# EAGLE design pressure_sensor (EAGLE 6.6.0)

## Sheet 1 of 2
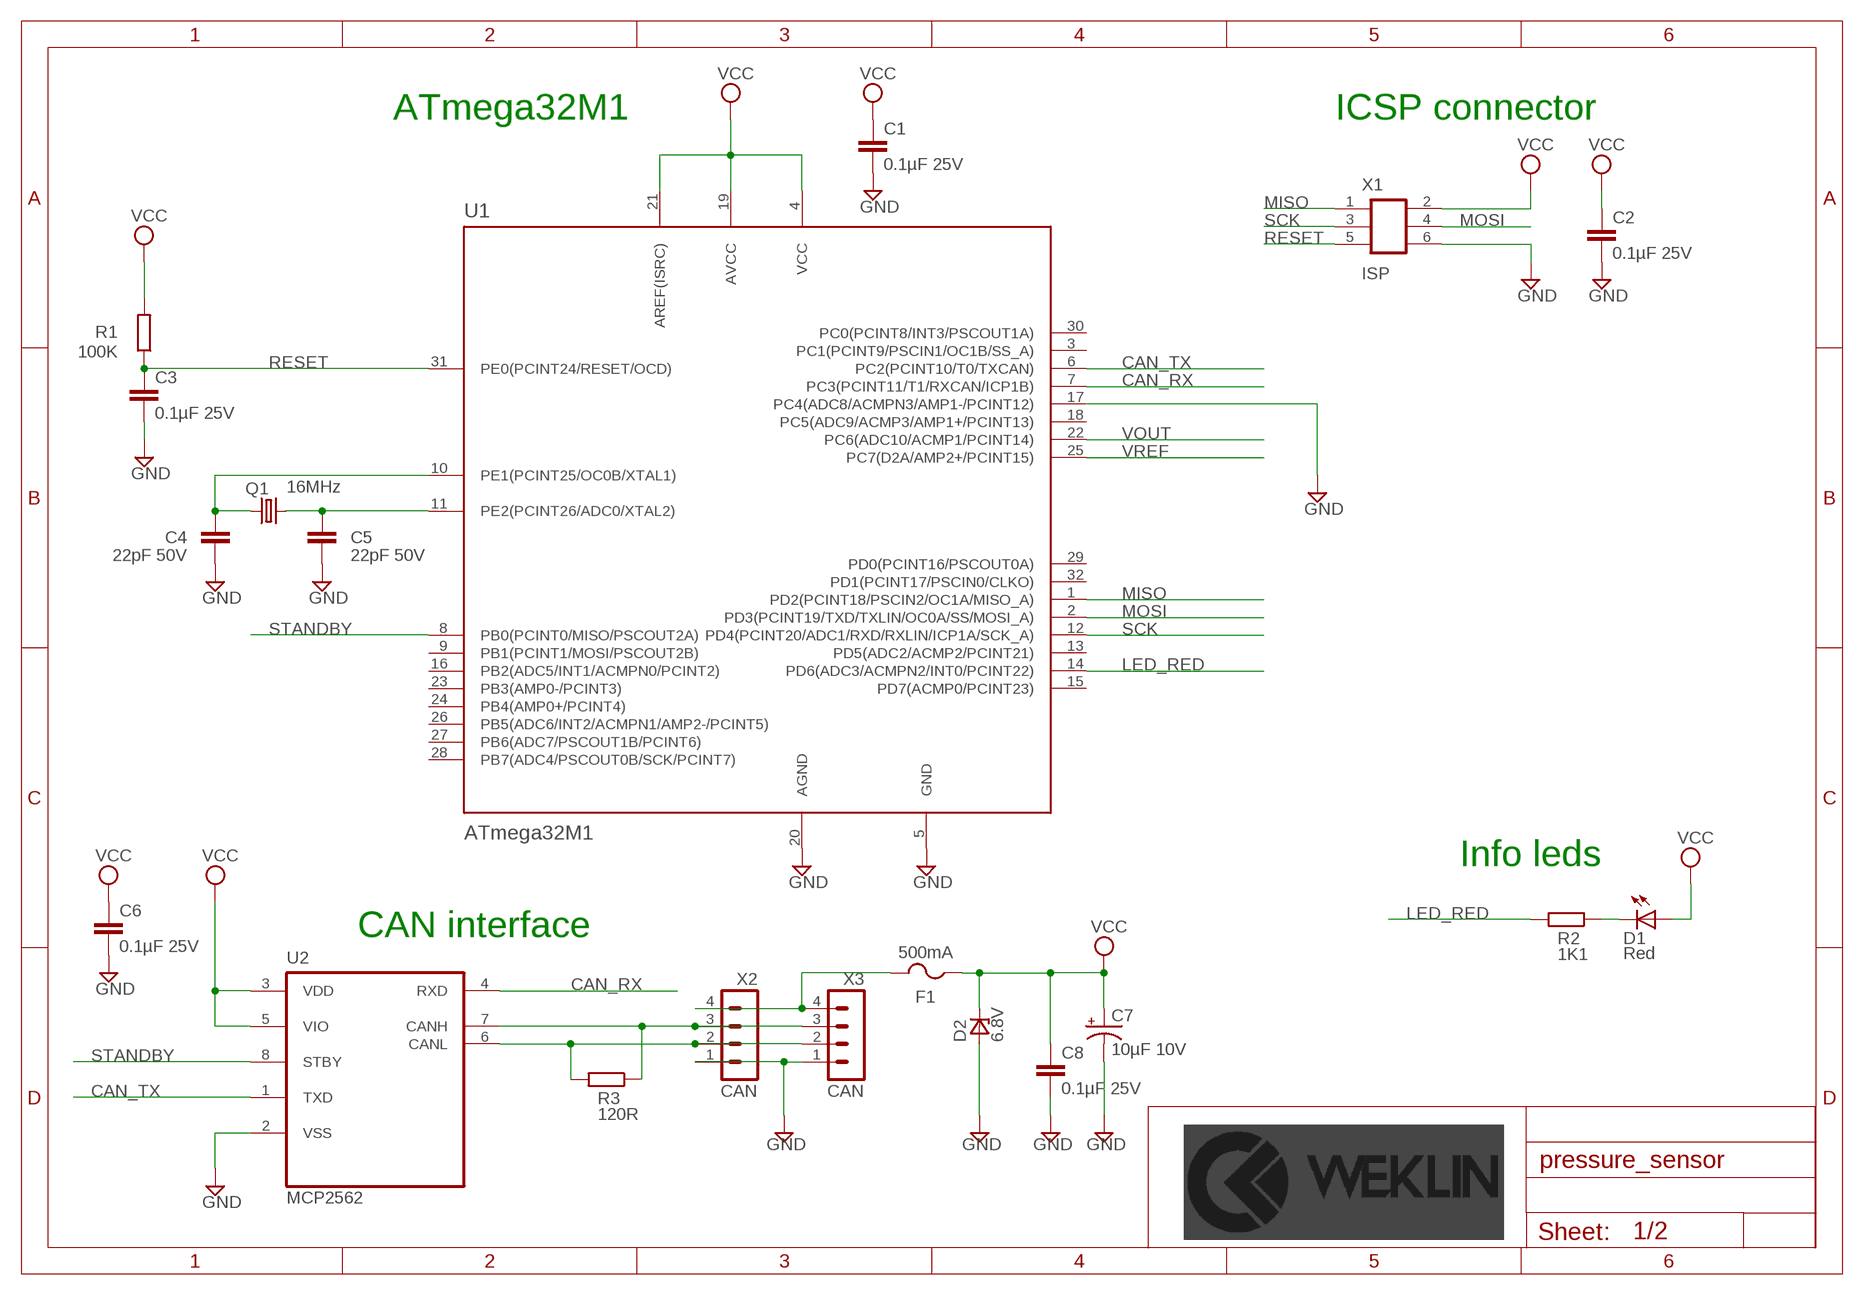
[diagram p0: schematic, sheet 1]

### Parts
C1  0.1µF 25V  CAPACITOR_NON_POL-100NF-25V(+-10%)(2012)  [C2012]
C2  0.1µF 25V  CAPACITOR_NON_POL-100NF-25V(+-10%)(2012)  [C2012]
C3  0.1µF 25V  CAPACITOR_NON_POL-100NF-25V(+-10%)(2012)  [C2012]
C4  22pF 50V  CAPACITOR_NON_POL-22PF-50V(+-5%)(2012)  [C2012]
C5  22pF 50V  CAPACITOR_NON_POL-22PF-50V(+-5%)(2012)  [C2012]
C6  0.1µF 25V  CAPACITOR_NON_POL-100NF-25V(+-10%)(2012)  [C2012]
C7  10µF 10V  CAPACITOR_POL-10µF-10V(+-10%)(3216)  [EIA3216]
C8  0.1µF 25V  CAPACITOR_NON_POL-100NF-25V(+-10%)(2012)  [C2012]
D1  Red  LEDVLDS1235G  [VLD]
D2  6.8V  ZENER_UNIDIR6.8  [DO-214AA]
F1  500mA  FUSE0451.500MRL  [EIARS-481-2]
Q1  16MHz  CRYSTAL-16MHZ_SMD(3225)  [SMD_KX7]
R1  100K  RESISTOR-100K(+-1%)(2012)  [R2012]
R2  1K1  RESISTOR-1K1(+-1%)(2012)  [R2012]
R3  120R  RESISTOR-120R(+-1%)(2012)  [R2012]
U1  ATmega32M1  ATMEGA32M1-TQFP32  [TQFP32]
U2  MCP2562  MCP2562-E/SN-SOIC8  [SOIC8]
X1  ISP  CON_2X3-SMD_1.27MM_MALE  [2X3_1.27MM_MALE_SMD]
X2  CAN  MICROLOCK-4CMS_HORIZONTAL  [504195-0470]
X3  CAN  MICROLOCK-4CMS_HORIZONTAL  [504195-0470]

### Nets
CAN_RX: U1.7(PC3(PCINT11/T1/RXCAN/ICP1B)) U2.4(RXD)
CAN_TX: U1.6(PC2(PCINT10/T0/TXCAN)) U2.1(TXD)
GND: C1.2 C2.2 C3.2 C4.2 C5.2 C6.2 C7.C(-) C8.2 D2.A U1.5(GND) U1.17(PC4(ADC8/ACMPN3/AMP1-/PCINT12)) U1.20(AGND) U2.2(VSS) X1.6 X2.1 X3.1 ; also sheet 2
LED_RED: R2.2 U1.14(PD6(ADC3/ACMPN2/INT0/PCINT22))
MISO: U1.1(PD2(PCINT18/PSCIN2/OC1A/MISO_A)) X1.1
MOSI: U1.2(PD3(PCINT19/TXD/TXLIN/OC0A/SS/MOSI_A)) X1.4
N$2: D1.C R2.1
N$4: F1.2 X2.4 X3.4
N$5: R3.2 U2.6(CANL) X2.2 X3.2
N$6: R3.1 U2.7(CANH) X2.3 X3.3
N$7: C5.1 Q1.3 U1.11(PE2(PCINT26/ADC0/XTAL2))
N$9: C4.1 Q1.1 U1.10(PE1(PCINT25/OC0B/XTAL1))
RESET: C3.1 R1.1 U1.31(PE0(PCINT24/RESET/OCD)) X1.5
SCK: U1.12(PD4(PCINT20/ADC1/RXD/RXLIN/ICP1A/SCK_A)) X1.3
STANDBY: U1.8(PB0(PCINT0/MISO/PSCOUT2A)) U2.8(STBY)
VCC: C1.1 C2.1 C6.1 C7.A(+) C8.1 D1.A D2.C F1.1 R1.2 U1.4(VCC) U1.19(AVCC) U1.21(AREF(ISRC)) U2.3(VDD) U2.5(VIO) X1.2 ; also sheet 2
VOUT: U1.22(PC6(ADC10/ACMP1/PCINT14)) ; also sheet 2
VREF: U1.25(PC7(D2A/AMP2+/PCINT15)) ; also sheet 2
Unconnected: U1.3(PC1(PCINT9/PSCIN1/OC1B/SS_A)) U1.9(PB1(PCINT1/MOSI/PSCOUT2B)) U1.13(PD5(ADC2/ACMP2/PCINT21)) U1.15(PD7(ACMP0/PCINT23)) U1.16(PB2(ADC5/INT1/ACMPN0/PCINT2)) U1.18(PC5(ADC9/ACMP3/AMP1+/PCINT13)) U1.23(PB3(AMP0-/PCINT3)) U1.24(PB4(AMP0+/PCINT4)) U1.26(PB5(ADC6/INT2/ACMPN1/AMP2-/PCINT5)) U1.27(PB6(ADC7/PSCOUT1B/PCINT6)) U1.28(PB7(ADC4/PSCOUT0B/SCK/PCINT7)) U1.29(PD0(PCINT16/PSCOUT0A)) U1.30(PC0(PCINT8/INT3/PSCOUT1A)) U1.32(PD1(PCINT17/PSCIN0/CLKO))

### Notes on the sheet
- ATmega32M1 | ICSP connector
- Info leds
- CAN interface

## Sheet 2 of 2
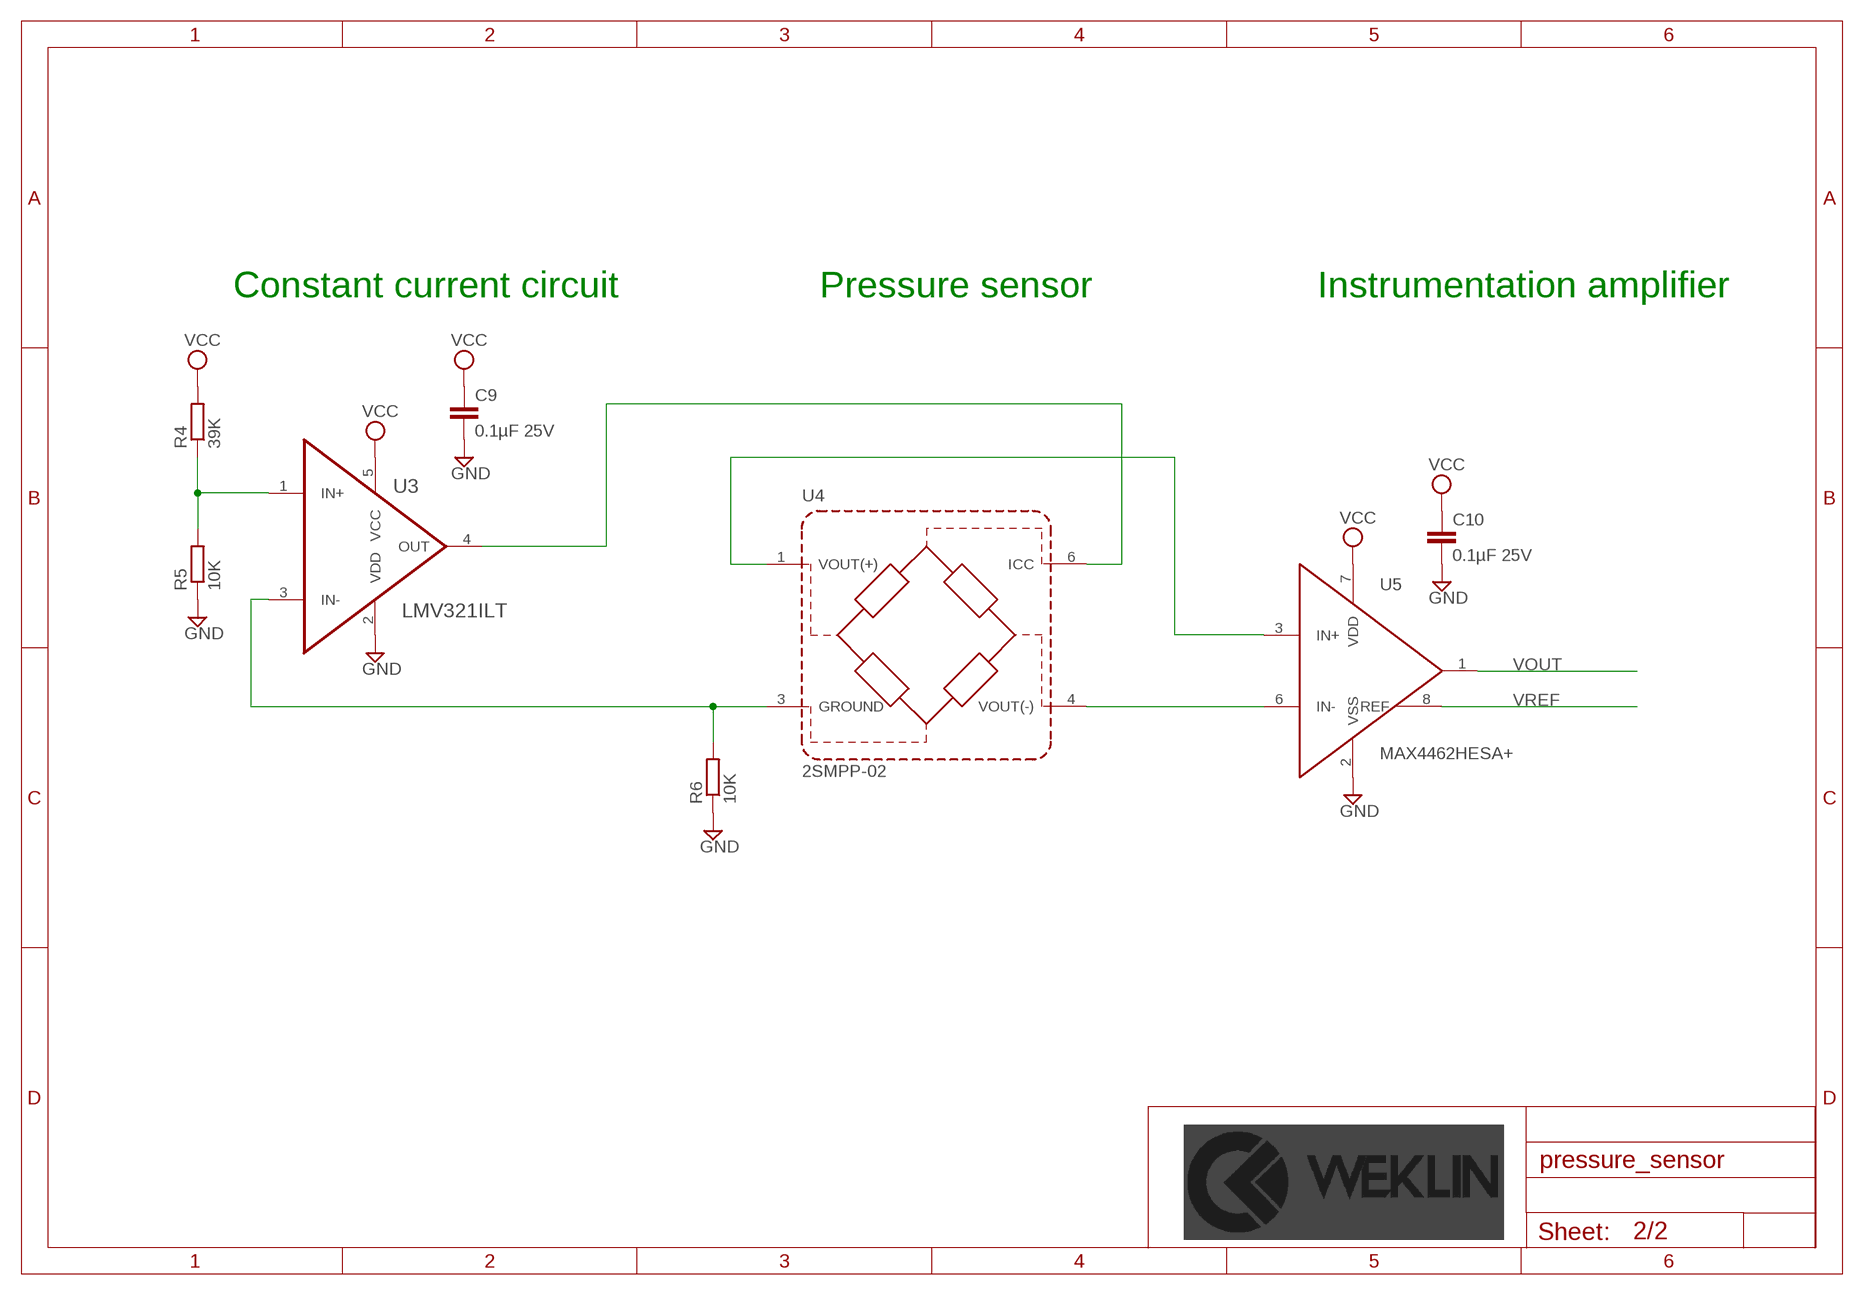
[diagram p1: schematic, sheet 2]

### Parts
C9  0.1µF 25V  CAPACITOR_NON_POL-100NF-25V(+-10%)(2012)  [C2012]
C10  0.1µF 25V  CAPACITOR_NON_POL-100NF-25V(+-10%)(2012)  [C2012]
R4  39K  RESISTOR-39K(+-1%)(2012)  [R2012]
R5  10K  RESISTOR-10K(+-1%)(2012)  [R2012]
R6  10K  RESISTOR-10K(+-1%)(2012)  [R2012]
U3  LMV321ILT  [SOT-23-5]
U4  2SMPP-02  2SMPP-03  [2SMPP-0X]
U5  MAX4462HESA+  [SOIC8]

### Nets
GND: C9.2 C10.2 R5.1 R6.1 U3.2(VDD) U5.2(VSS) ; also sheet 1
N$1: U4.4(VOUT(-)) U5.6(IN-)
N$3: U4.1(VOUT(+)) U5.3(IN+)
N$8: U3.4(OUT) U4.6(ICC)
N$10: R4.1 R5.2 U3.1(IN+)
N$15: R6.2 U3.3(IN-) U4.3(GROUND)
VCC: C9.1 C10.1 R4.2 U3.5(VCC) U5.7(VDD) ; also sheet 1
VOUT: U5.1(OUT) ; also sheet 1
VREF: U5.8(REF) ; also sheet 1
Unconnected: U4.2(NC) U4.5(N-SUB)

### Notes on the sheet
- Constant current circuit | Pressure sensor | Instrumentation amplifier

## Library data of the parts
C1-C3 C6 C8-C10 = weklin_capacitor:CAPACITOR_NON_POL: Condensateur céramique multicouche; LIB: weklin_capacitor; MANUFACTURER: AVX; MPN: 08053C104KAT2A; OC_FARNELL: 2280951; PRICE: 0,0036
C4 C5 = weklin_capacitor:CAPACITOR_NON_POL: Condensateur céramique multicouche; LIB: weklin_capacitor; MANUFACTURER: Multicomp; MPN: MC0805N220J500CT; OC_FARNELL: 2310684; PRICE: 0,0078
C7 = weklin_capacitor:CAPACITOR_POL: Capacitor; LIB: weklin_capacitor; MANUFACTURER: Kemet; MPN: T491A106K010AT; OC_FARNELL: 2250086; PRICE: 0,0578
D1 = weklin_led:LED: Led; LIB: weklin_led; MANUFACTURER: Vishay; MPN: VLDS1235G; OC_FARNELL: 2494682; PRICE: 0,003
D2 = weklin_diode:ZENER_UNIDIR: P6SMBxxA Series of unidirectional Transient Voltage Suppressor Diodes; LIB: weklin_diode; MANUFACTURER: ON Semiconductor; MPN: P6SMB6.8AT3G; OC_FARNELL: 1459166RL; PRICE: 0,178
F1 = weklin_fuse:FUSE: Fuse; LIB: weklin_fuse; MANUFACTURER: Littlefuse; MPN: 0451500MRL; OC_FARNELL: 2383271; PRICE: 0,527
Q1 = weklin_crystal:CRYSTAL: Crystal resonator; LIB: weklin_crystal; MANUFACTURER: AEL CRYSTALS; MPN: E3SB16.0000F09G11AE; OC_FARNELL: 2467444RL; PRICE: 0,315
R1 = weklin_resistor:RESISTOR: Resistor; LIB: weklin_resistor; MANUFACTURER: Multicomp; MPN: MCWR08X1003FTL; OC_FARNELL: 2446868; PRICE: 0,0014
R2 = weklin_resistor:RESISTOR: Resistor; LIB: weklin_resistor; MANUFACTURER: Multicomp; MPN: MC0805S8F1101T5E; OC_FARNELL: 1635316; PRICE: 0,003
R3 = weklin_resistor:RESISTOR: Resistor; LIB: weklin_resistor; MANUFACTURER: Multicomp; MPN: MCWR08X1200FTL; OC_FARNELL: 2446878; PRICE: 0,0014
R4 = weklin_resistor:RESISTOR: Resistor; LIB: weklin_resistor; MANUFACTURER: Multicomp; MPN: MC01W0805139K; OC_FARNELL: 2129244; PRICE: 0,001
R5 R6 = weklin_resistor:RESISTOR: Resistor; LIB: weklin_resistor; MANUFACTURER: Multicomp; MPN: MCWR08X1002FTL; OC_FARNELL: 2446870; PRICE: 0,0014
U1 = weklin_micro-atmell:ATMEGA32M1: ATMEL ATMEGA32M1-AU MCU 8 BITS ATMEGA 16MHZ; LIB: weklin_micro_atmell; MANUFACTURER: Atmel; MPN: ATmega32M1-AU; OC_FARNELL: 2443180; PRICE: 6,18
U2 = weklin_ic_can:MCP2562-E/SN: High-Speed CAN Transceiver; LIB: weklin_ic_can; MANUFACTURER: Microchip; MPN: MCP2562-E/SN; OC_FARNELL: 2362839; PRICE: 1,12
U3 = weklin_amplifier:LMV321ILT: operational amplifiers,SOT23-5; LIB: weklin_amplifier; MANUFACTURER: ST Microelectronics; MPN: LMV321ILT; OC_FARNELL: 2253412; PRICE: 0,156
U4 = weklin_sensor:2SMPP: OMRON - MEMS Gauge pressure Sensor 2SMPP; LIB: weklin_sensor; MANUFACTURER: Omron; MPN: 2SMPP-03; OC_FARNELL: 2293688; PRICE: 4,31
U5 = weklin_amplifier:MAX4462: Low Cost, Low Power, Instrumentation Amplifier Source: http://www.analog.com/UploadedFiles/Data_Sheets/37793330023930AD620_e.pdf; LIB: weklin_amplifier; MANUFACTURER: Maxim; MPN: MAX4462HESA+; OC_FARNELL: 2516876; PRICE: 3,06
X1 = weklin_connector:CON_2X3: Board-To-Board Connector, Micro-MaTch Series, Embase, 6voies.; LIB: weklin_connector; MANUFACTURER: Minitek; MPN: 20021121-00006C4LF; OC_FARNELL: 1865277; PRICE: 0,333
X2 X3 = weklin_micro-lock:MICROLOCK-4: Connecteur MOLEX de 4 Contacts Série Mini50 GEII/IUT ANGERS; LIB: weklin_micro-lock; MANUFACTURER: Molex; MPN: 504195-0470; OC_FARNELL: 2445490; PRICE: 0,713

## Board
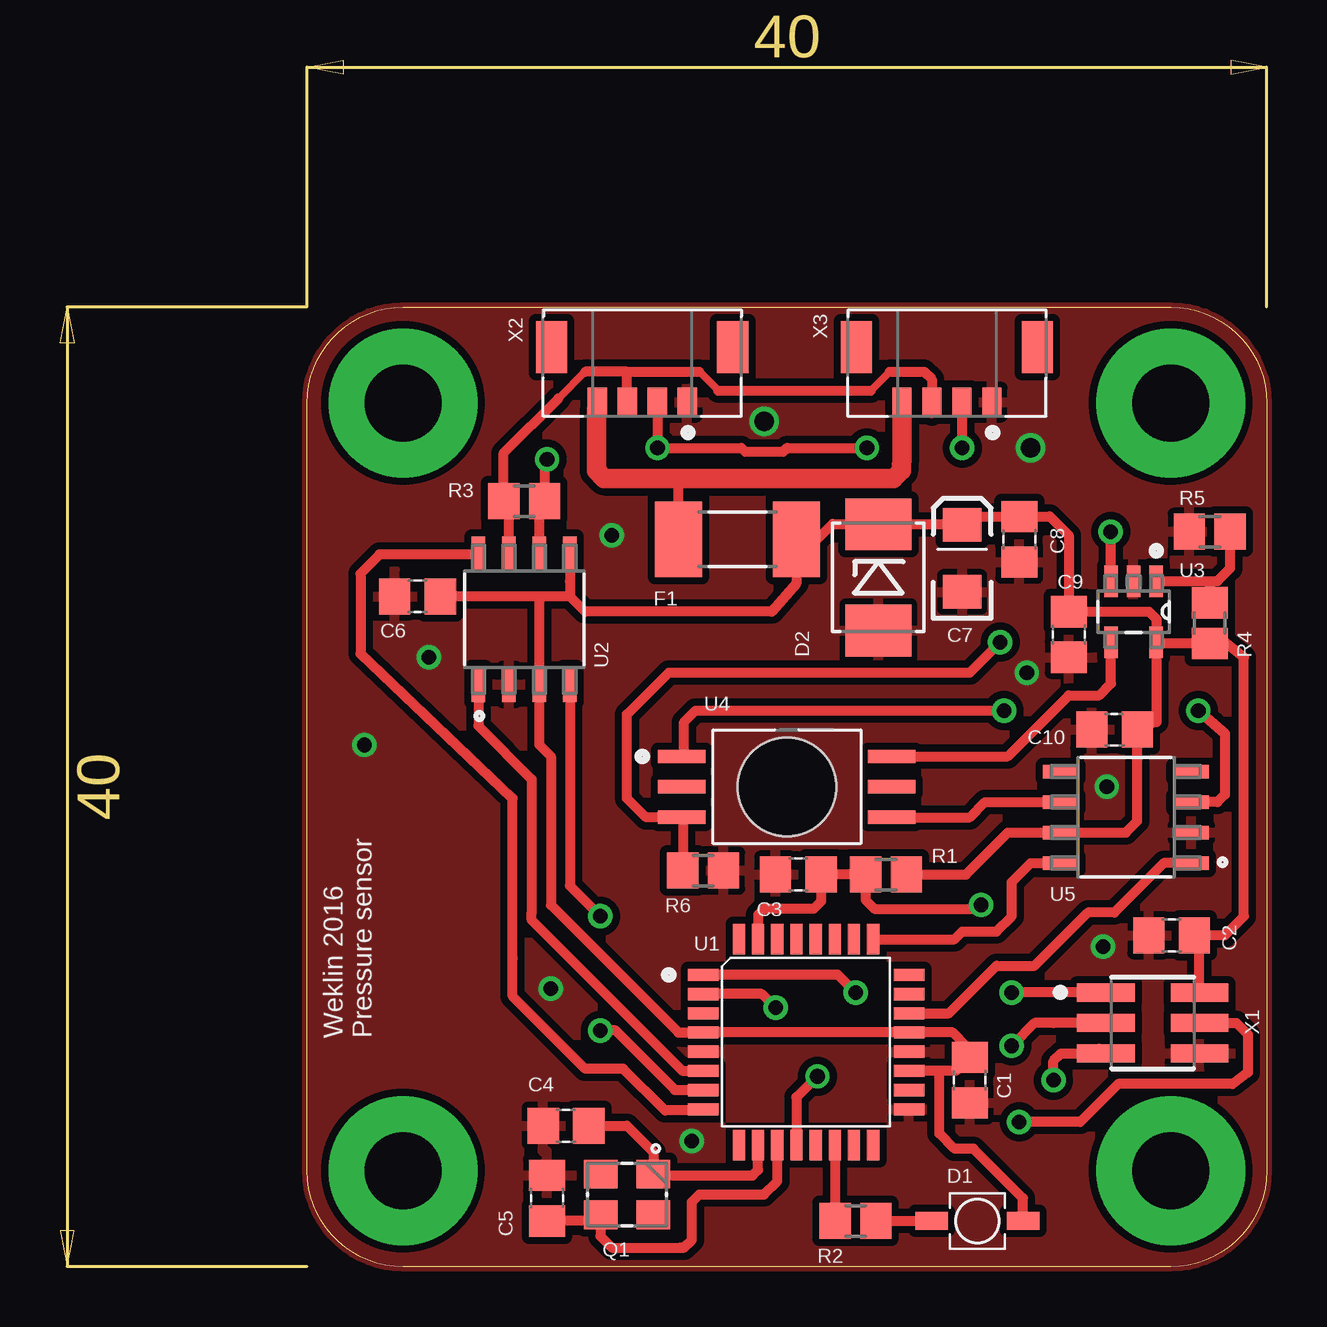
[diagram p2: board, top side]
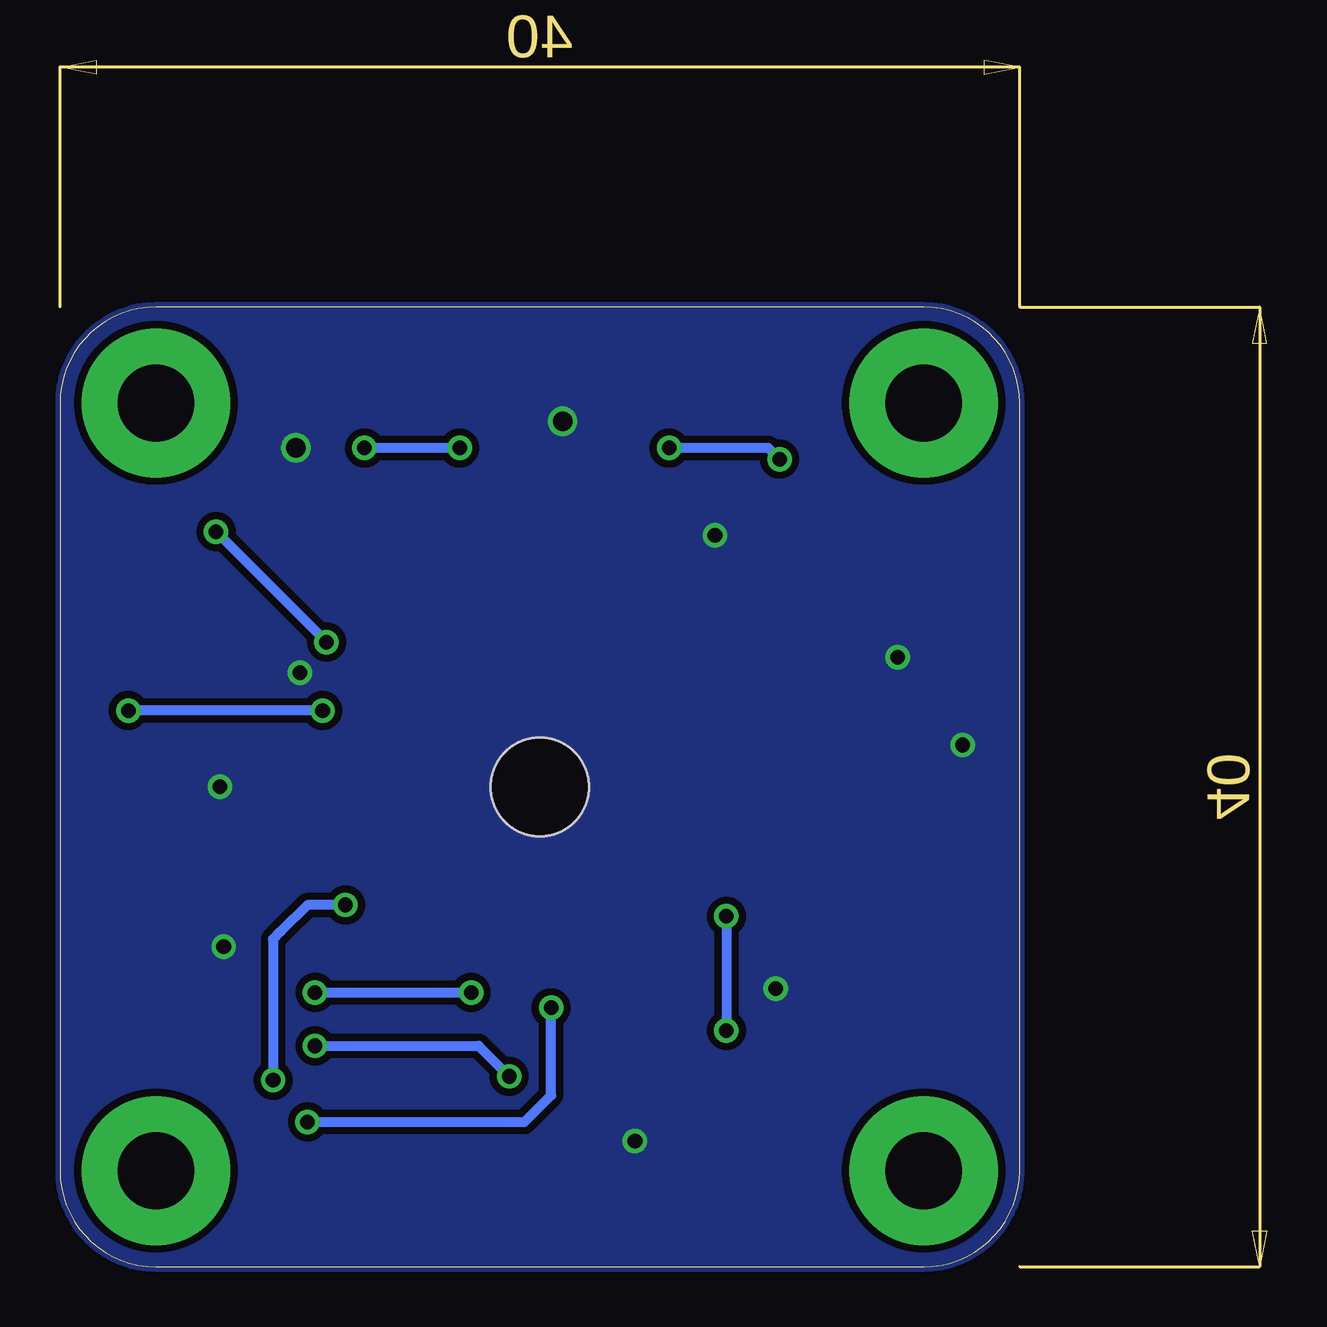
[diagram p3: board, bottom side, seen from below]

Size 50.3 x 50.3 mm. Coordinates in mm from the lower left corner, seen from the top.
Outline: 10.3,4 10.3,36 arc-90 14.3,40 46.3,40 arc-90 50.3,36 50.3,4 arc-90 46.3,0 14.3,0 arc-90 10.3,4
Copper layers (1*16): Top 0.035mm / dielectric 1.5mm / Bottom 0.035mm
Design rules "default *": minimum track width 10mil, minimum drill 24mil, track to track 12mil, track to pad 12mil, pad to pad 8mil, via to via 8mil, smd to smd 8mil, copper to edge 0mil, drill to drill 8mil, minimum pad ring 10mil, minimum via ring 8mil, stop-mask expansion 4mil, vias tented up to drill 0mil, thermal gap 10mil

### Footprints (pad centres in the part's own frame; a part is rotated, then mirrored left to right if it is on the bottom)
C2012 = smd 1.3 x 1.5: 1 -0.95,0; 2 0.95,0
EIA3216 = smd 1.4 x 1.6: A 1.4,0; C -1.4,0
VLD = smd 1.35 x 0.75: A 1.9,0; C -1.9,0
DO-214AA = smd 2.159 x 2.743: A 2.21,0; C -2.21,0
EIARS-481-2 = smd 1.956 x 3.15: 1 -2.451,0; 2 2.451,0
SMD_KX7 = smd 1.4 x 1.2: 1 -1.1,-0.85; 2 1.1,-0.85; 3 1.1,0.85; 4 -1.1,0.85
R2012 = smd 1.3 x 1.5: 1 -0.85,0; 2 0.85,0
TQFP32 = smd 1.27 x 0.508: 1 -4.293,2.8; 2 -4.293,2; 3 -4.293,1.2; 4 -4.293,0.4; 5 -4.293,-0.4; 6 -4.293,-1.2; 7 -4.293,-2; 8 -4.293,-2.8; 17 4.293,-2.8; 18 4.293,-2; 19 4.293,-1.2; 20 4.293,-0.4; 21 4.293,0.4; 22 4.293,1.2; 23 4.293,2; 24 4.293,2.8 | smd 0.508 x 1.27: 9 -2.8,-4.293; 10 -2,-4.293; 11 -1.2,-4.293; 12 -0.4,-4.293; 13 0.4,-4.293; 14 1.2,-4.293; 15 2,-4.293; 16 2.8,-4.293; 25 2.8,4.293; 26 2,4.293; 27 1.2,4.293; 28 0.4,4.293; 29 -0.4,4.293; 30 -1.2,4.293; 31 -2,4.293; 32 -2.8,4.293
SOIC8 = smd 1.473 x 0.559: 1 -2.718,1.905; 2 -2.718,0.635; 3 -2.718,-0.635; 4 -2.718,-1.905; 5 2.718,-1.905; 6 2.718,-0.635; 7 2.718,0.635; 8 2.718,1.905
SOT-23-5 = smd 1.321 x 0.559: 1 -1.27,0.94; 2 -1.27,0; 3 -1.27,-0.94; 4 1.27,-0.94; 5 1.27,0.94
2SMPP-0X = smd 1.981 x 0.559: 1 -4.375,1.27; 2 -4.375,0; 3 -4.375,-1.27; 4 4.375,-1.27; 5 4.375,0; 6 4.375,1.27 | hole 4.1: 0,0
2X3_1.27MM_MALE_SMD = smd 2.4 x 0.76: 1 -1.95,1.27; 2 1.95,1.27; 3 -1.95,0; 4 1.95,0; 5 -1.95,-1.27; 6 1.95,-1.27
504195-0470 = smd 0.8 x 1.2: 1 1.875,0; 2 0.625,0; 3 -0.625,0; 4 -1.875,0 | smd 1.3 x 2.15: P$5 -3.775,2.295; P$6 3.775,2.295

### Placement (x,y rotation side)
C1  37.92,7.78 270 top
C2  46.34,13.81 180 top
C3  30.78,16.35 180 top
C4  21.09,5.87 180 top
C5  20.3,2.86 90 top
C6  14.9,27.94 180 top
C7  37.61,29.53 90 top
C8  39.99,30.32 270 top
C9  42.05,26.35 270 top
C10  43.95,22.38 180 top
D1  38.24,1.91 0 top
D2  34.11,28.73 270 top
DRILEGEND  [DRILEGEND]  not placed on the board
F1  28.24,30.32 180 top
Q1  23.64,3.02 180 top
R1  34.43,16.35 0 top
R2  33.16,1.91 180 top
R3  19.35,31.91 0 top
R4  47.92,26.83 270 top
R5  47.92,30.64 0 top
R6  26.81,16.51 180 top
U1  31.1,9.37 0 top
U2  19.35,26.99 90 top
U3  44.75,27.3 270 top
U4  30.3,20 0 top
U5  44.43,18.73 180 top
X1  45.54,10.16 0 top
X2  24.27,36.04 0 top
X3  36.97,36.04 0 top

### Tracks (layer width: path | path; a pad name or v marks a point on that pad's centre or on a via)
CAN_RX  (via drill 0.61)
  Top 0.406: U2.4 21.25,15.88 v22.52,14.61 | U1.7 25.64,7.37 23.16,9.84 v22.52,9.84
  Bottom 0.406: v22.52,14.61 v22.52,9.84
CAN_TX
  Top 0.406: U2.1 17.44,22.54 19.67,20.32 19.67,14.76 19.67,14.45 25.95,8.17 U1.6
GND  (via drill 0.61, 0.81)
  other vias: 15.38,25.4 12.68,21.75 29.35,35.24 26.33,5.24 43.64,20 43.48,13.34 40.3,24.77 20.46,11.59 23,30.48 40.46,34.13
  pour Bottom: 10.3,4 10.3,36 arc-90 14.3,40 46.3,40 arc-90 50.3,36 50.3,4 arc-90 46.3,0 14.3,0 arc-90
  pour Top: 10.3,4 10.3,36 arc-90 14.3,40 46.3,40 arc-90 50.3,36 50.3,4 arc-90 46.3,0 14.3,0 arc-90
LED_RED
  Top 0.406: U1.14 R2.2
MISO  (via drill 0.61)
  Top 0.406: X1.1 v39.67,11.43 | v33.16,11.43 32.42,12.17 U1.1
  Bottom 0.406: v39.67,11.43 v33.16,11.43
MOSI  (via drill 0.61)
  Top 0.406: X1.4 49.03,10.16 49.51,9.68 49.51,8.1 48.88,7.62 44.11,7.62 42.53,6.03 v39.99,6.03 | v29.83,10.79 29.25,11.37 U1.2
  Bottom 0.406: v39.99,6.03 30.94,6.03 29.83,7.14 v29.83,10.79
N$1
  Top 0.406: U4.4 37.92,18.73 38.56,19.37 U5.6
N$2
  Top 0.406: R2.1 D1.C
N$3  (via drill 0.61)
  Top 0.406: U4.1 26.02,21.36 26.02,22.7 26.49,23.18 v39.35,23.18 | v47.45,23.18 48.56,22.23 48.56,19.68 48.24,19.37 U5.3
  Bottom 0.406: v39.35,23.18 v47.45,23.18
N$4
  Top 0.406: F1.2 25.79,32.61 25.7,32.86
  Top 0.813: X2.4 22.37,35.56 22.37,33.18 22.68,32.86 25.7,32.86 34.75,32.86 35.06,33.18 35.09,33.84 X3.4
N$5  (via drill 0.61)
  Top 0.406: v37.61,34.13 37.61,35.55 X3.2 | v20.3,33.66 20.2,33.55 R3.2 19.98,31.91 U2.6 | v33.64,34.13 30.3,34.13 30.14,33.97 28.56,33.97 28.4,34.13 v24.91,34.13 24.91,36.03 X2.2
  Bottom 0.406: v24.91,34.13 21.27,34.13 20.78,34.13 v20.3,33.66 | v33.64,34.13 v37.61,34.13
N$6
  Top 0.305: 26.65,37.31 27.45,36.51 | 33.8,36.51 34.59,37.31 | 21.89,37.31 20.78,36.2
  Top 0.406: X2.3 23.65,36.52 23.64,37.31 | 23.64,37.31 26.65,37.31 | X3.3 36.34,35.57 36.34,36.99 36.02,37.31 34.59,37.31 | U2.7 18.71,31.91 R3.1 18.5,33.92 20.78,36.2 | 27.45,36.51 33.8,36.51 | 23.64,37.31 21.89,37.31
N$7
  Top 0.406: 22.52,2.15 Q1.3 22.52,2.15 | 22.52,2.15 22.52,1.27 23,0.79 25.86,0.79 26.02,0.79 26.33,1.11 26.33,2.06 26.33,2.7 26.65,3.02 29.35,3.02 29.9,3.56 U1.11 | 22.52,2.15 22.28,1.91 C5.1
N$8
  Top 0.406: U4.6 39.51,21.27 42.05,23.81 43.32,23.81 43.81,24.3 U3.4
N$9
  Top 0.406: U1.10 29.1,4.03 28.87,3.81 27.29,3.81 26.81,3.81 24.79,3.81 Q1.1 24.73,4.77 23.64,5.87 C4.1
N$10
  Top 0.406: U3.1 48.14,28.57 | 48.14,28.57 48.24,28.57 48.72,29.05 48.77,29.11 R5.2 | 48.14,28.57 47.92,28.47 R4.1
N$11  (via drill 3.2 pad 6.2)
  other vias: 14.3,36
N$12  (via drill 3.2 pad 6.2)
  other vias: 46.3,36
N$13  (via drill 3.2 pad 6.2)
  other vias: 46.3,4
N$14  (via drill 3.2 pad 6.2)
  other vias: 14.3,4
N$15  (via drill 0.61)
  Top 0.406: U3.3 43.81,30.63 v43.8,30.64 | U4.3 | U4.3 25.96,18.7 R6.2 | U4.3 24.43,18.73 23.64,19.53 23.64,23.02 25.38,24.77 37.92,24.77 v39.19,26.04
  Bottom 0.406: v39.19,26.04 v43.8,30.64
RESET  (via drill 0.61)
  Top 0.406: U1.31 29.1,14.67 29.19,14.76 29.35,14.92 31.41,14.92 31.73,15.24 C3.1 R1.1 33.58,15.3 33.95,14.92 38.24,14.92 v38.4,15.08 | 43.32,9.09 X1.5 41.73,8.89 41.41,8.57 v41.41,7.78
  Bottom 0.406: v38.4,15.08 39.99,15.08 41.1,13.97 41.41,13.65 41.41,8.1 v41.41,7.78
SCK  (via drill 0.61)
  Top 0.406: X1.3 41.41,10.16 40.62,10.16 v39.67,9.21 | v31.57,7.94 30.7,7.06 U1.12
  Bottom 0.406: v39.67,9.21 32.84,9.21 v31.57,7.94
STANDBY
  Top 0.406: U2.8 17.43,29.69 13.32,29.69 12.52,28.89 12.52,25.56 18.87,19.53 18.87,12.86 18.87,11.27 21.89,8.26 23.48,8.26 25.22,6.51 26.75,6.51 U1.8
VCC
  Top 0.406: U2.5 21.25,28.57 21.25,27.94 19.98,27.94 | 19.98,27.94 C6.1 | 19.98,27.78 U2.3 19.98,21.75 20.46,21.27 20.46,15.08 25.77,9.77 U1.4 U1.21 37.21,9.77 37.76,9.21 37.92,9.05 C1.1 37.36,8.17 36.58,8.17 | 19.98,27.78 19.98,27.94 | 19.98,27.78 20.14,27.94 21.25,27.94 21.89,27.3 29.67,27.3 30.69,28.49 F1.1 31.57,30.32 32.21,30.96 34.1,30.96 D2.C 34.13,30.93 C7.A 37.95,31.27 C8.1 41.26,31.27 42.05,30.48 C9.1 45.39,27.3 45.7,26.99 45.7,26.05 U3.5 45.75,25.98 | 45.75,25.98 R4.2 48.61,25.98 49.35,25.4 49.35,14.61 48.56,13.81 C2.1 46.97,13.97 47.49,13.97 | 45.75,25.98 45.7,25.93 45.7,22.7 C10.1 44.91,18.57 44.43,18.1 U5.7 39.51,18.1 37.76,16.35 R1.2 | D1.A 40.14,2.86 38.08,4.92 37.29,4.92 36.65,5.56 36.65,8.1 36.58,8.17 | X1.2 47.49,13.97 | 47.49,13.97 47.49,14.33 | U1.19 36.18,8.17 36.27,8.17 36.49,8.17 36.58,8.17
VOUT
  Top 0.406: U1.22 37.06,10.57 39.03,12.54 40.62,12.54 42.84,14.76 43.95,14.76 46.02,16.83 U5.1
VREF
  Top 0.406: U1.25 37.29,13.65 37.61,13.97 39.03,13.97 39.67,14.61 39.67,16.03 40.46,16.83 U5.8

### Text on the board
tPlace: Weklin 2016 / Pressure sensor
DrillLegend: LAYER-STACK
DrillLegend_01-16: 01-16
DrillLegend_01-20: 01-20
